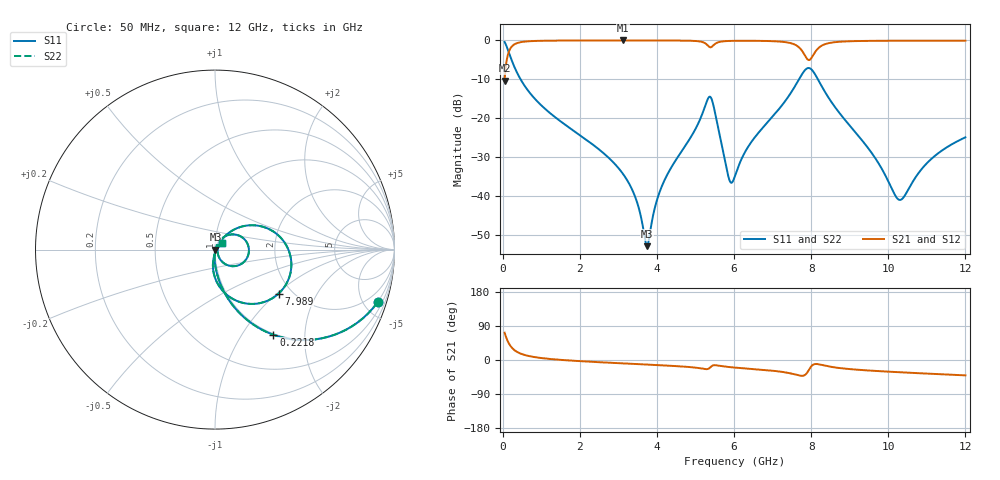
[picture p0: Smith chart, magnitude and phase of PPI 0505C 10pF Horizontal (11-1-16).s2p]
# MHz S MA R 50
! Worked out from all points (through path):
!   1601 points, 50 MHz to 12 GHz, reference 50 ohm
!   highest |S21| = -0.02 dB at 3.12 GHz (marker M1); lowest = -10.3 dB at 50 MHz (marker M2)
!   group delay of S21, straight-line fit = 11.7 ps
!   lowest |S11| = -52.9 dB at 3.74 GHz (marker M3), VSWR 1.00, Z = 50.2 - j0.0645 ohm
!   |S11| at or under -10 dB: 463.8 MHz to 7.685 GHz (7.221 GHz wide, 177 % of centre); 8.175 GHz to end of sweep
!   |S22| runs from -52.9 to -0.4 dB; largest |S21 - S12| = 0
!   S11 on the Smith chart (normalised r, x): 50 MHz: 0.98, -6.20; 221.8 MHz: 0.98, -1.39; 7.989 GHz: 1.71, -1.03; 12 GHz: 1.08, +0.08
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50  0.9525 -17.9  0.3044 72.1  0.3044 72.1  0.9525 -17.9
221.7812  0.5752 -55.6  0.8175 34.4  0.8175 34.4  0.5752 -55.6
625.0938  0.238 -78.1  0.9705 11.7  0.9705 11.7  0.238 -78.1
2044.156  0.05849 -91.9  0.9968 -3.2  0.9968 -3.2  0.05849 -91.9
3119.656  0.01925 -93.6  0.9978 -9.0  0.9978 -9.0  0.01925 -93.6
3455.75  0.009177 -87.9  0.9977 -10.6  0.9977 -10.6  0.009177 -87.9
3739.562  0.002268 -16.4  0.9975 -12.0  0.9975 -12.0  0.002268 -16.4
4038.312  0.01015 61.2  0.997 -13.5  0.997 -13.5  0.01015 61.2
5360.281  0.1885 2.1  0.8241 -21.5  0.8241 -21.5  0.1885 2.1
5472.312  0.1413 -40.9  0.8718 -13.8  0.8718 -13.8  0.1413 -40.9
5868.156  0.01671 -30.0  0.9832 -18.6  0.9832 -18.6  0.01671 -30.0
6025  0.0181 27.5  0.9873 -20.0  0.9873 -20.0  0.0181 27.5
6405.906  0.04607 54.4  0.9886 -23.0  0.9886 -23.0  0.04607 54.4
7615.844  0.2757 28.8  0.8623 -39.0  0.8623 -39.0  0.2757 28.8
7854.844  0.4223 -5.1  0.6189 -38.3  0.6189 -38.3  0.4223 -5.1
7989.281  0.431 -34.6  0.5783 -18.4  0.5783 -18.4  0.431 -34.6
8019.156  0.4178 -40.9  0.6071 -14.9  0.6071 -14.9  0.4178 -40.9
8459.812  0.1807 -86.8  0.9227 -17.0  0.9227 -17.0  0.1807 -86.8
10013.31  0.01498 -79.4  0.9894 -30.8  0.9894 -30.8  0.01498 -79.4
10341.94  0.009034 -18.3  0.9906 -32.6  0.9906 -32.6  0.009034 -18.3
11058.94  0.0282 38.7  0.9916 -36.1  0.9916 -36.1  0.0282 38.7
12000  0.05681 42.8  0.9911 -40.6  0.9911 -40.6  0.05681 42.8
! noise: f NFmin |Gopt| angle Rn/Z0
50  0.0004011  0.874  1.871  0.0006863
1372  0.003981  0.6739  4.896  0.002348
2701  0.006715  0.6302  8.912  0.003388
4031  0.01049  0.6449  12.9  0.005524
5360  0.1044  0.9443  17.16  0.4102
6682  0.0277  0.7639  21.16  0.02304
8012  0.2222  0.9611  25.42  1.227
9341  0.0372  0.7593  29.56  0.0293
1.067e+04  0.02895  0.6683  33.36  0.01544
1.2e+04  0.02796  0.6275  36.98  0.01272
